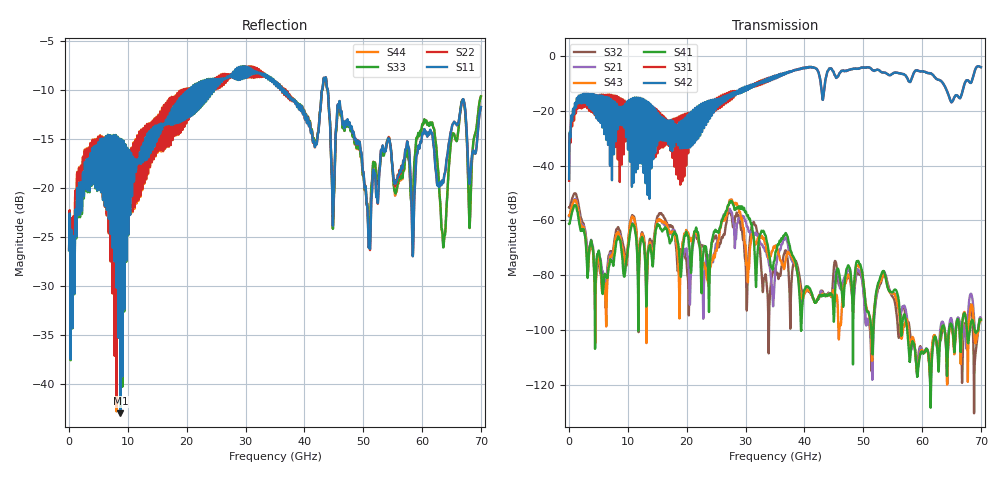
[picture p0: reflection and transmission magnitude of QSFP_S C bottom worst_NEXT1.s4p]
! AWR Design Environment (8415) Tue Jan 08 12:51:46 2019
! Document = 'QSFP Channel_S'
! nPorts: 4, nXvals: 7001
# HZ S DB R 50
!Freq DBS11 AngS11 DBS12 AngS12 DBS13 AngS13 DBS14 AngS14
!	DBS21 AngS21 DBS22 AngS22 DBS23 AngS23 DBS24 AngS24
!	DBS31 AngS31 DBS32 AngS32 DBS33 AngS33 DBS34 AngS34
!	DBS41 AngS41 DBS42 AngS42 DBS43 AngS43 DBS44 AngS44
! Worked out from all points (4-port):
!   7000 points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, 10 MHz to 70 GHz, reference 50 ohm
!   strongest paths, dB at 10 MHz, 17.51 GHz, 35.01 GHz, 52.51 GHz, 70 GHz:
!     S42: -44.9, -33.8, -7.3, -5.0, -4.0
!     S31: -45.5, -26.4, -7.4, -5.0, -4.0
!     S41: -61.3, -66.3, -73.3, -83.1, -96.3
!     S43: -58.3, -64.5, -69.5, -83.8, -96.5
!     S21: -58.6, -64.0, -79.9, -84.3, -95.7
!     S32: -55.3, -62.3, -77.9, -85.1, -96.0
!   lowest |S11| = -43.0 dB at 8.74 GHz (marker M1), VSWR 1.01, Z = 50.7 + j0.249 ohm
!   |S11| at or under -10 dB: start of sweep to 20.44 GHz; 36.44 GHz to 43.03 GHz (6.585 GHz wide, 16.6 % of centre); 43.97 GHz to end of sweep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
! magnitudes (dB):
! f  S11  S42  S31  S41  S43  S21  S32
! 10 MHz  -26.4  -44.9  -45.5  -61.3  -58.3  -58.6  -55.3
! 5.73 GHz  -19.2  -17.7  -18.6  -86.8  -85.2  -79.1  -79.5
! 8.74 GHz  -43.0  -20.2  -16.2  -68.0  -66.6  -65.8  -64.5
! 23.62 GHz  -10.8  -23.7  -21.9  -77.5  -82.8  -72.8  -79.4
! 27.53 GHz  -8.6  -13.7  -13.6  -53.2  -52.4  -56.9  -57.8
! 30.38 GHz  -8.7  -12.4  -11.9  -58.1  -82.2  -62.5  -77.2
! 70 GHz  -11.8  -4.0  -4.0  -96.3  -96.5  -95.7  -96.0
